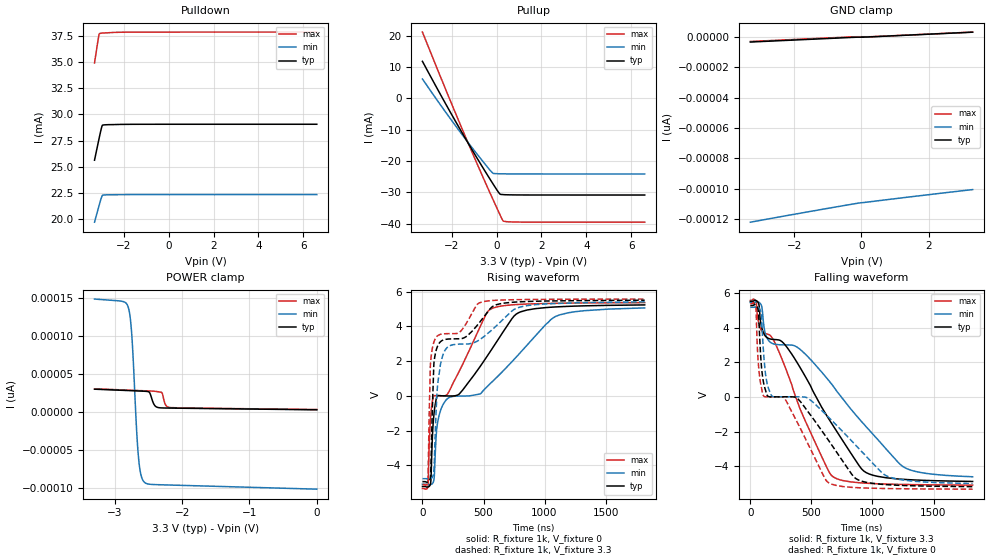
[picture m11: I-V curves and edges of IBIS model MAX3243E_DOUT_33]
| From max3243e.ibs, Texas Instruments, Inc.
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[Model]   MAX3243E_DOUT_33
Model_type  3-state
Enable   Active-High
Vref =   0
Rref =   3000
Cref =   150p
Vmeas =   1.5
| variable   typ   min   max
C_comp   3.62pF   2.98pF   4.25pF
| C_pullup   4.04pF   3.07pF   5.16pF
| C_pulldown   3.89pF   2.76pF   5.21pF
| C_tri-state   3.62pF   2.98pF   4.25pF
[Temperature Range]   40   100   -40
| Ambient temperature   25   85   -40
[Voltage range]   3.3   3   3.6
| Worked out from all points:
|   slope of the pullup table from 0 to 0.495 V, typ, clamps not added: 285 ohm
|   rising waveform, R_fixture 1k, V_fixture 0: 20-80 % time 533ns typ, 764ns min, 370ns max; typ from -5.23 V to 5.24 V
|   falling waveform, R_fixture 1k, V_fixture 3.3: 20-80 % time 648ns typ, 926ns min, 377ns max; typ from 5.53 V to -4.89 V
|   rising waveform, R_fixture 1k, V_fixture 3.3: 20-80 % time 285ns typ, 394ns min, 70.2ns max; typ from -4.95 V to 5.51 V
|   falling waveform, R_fixture 1k, V_fixture 0: 20-80 % time 619ns typ, 784ns min, 449ns max; typ from 5.29 V to -5.19 V
[GND Clamp]
| MAX3243E_DOUT_33
|   Voltage   I(typ)   I(min)   I(max)
-3.3V     -3.406pA   -122.2pA   -3.03pA
-1.41V    -1.49pA    -114.6pA   -1.116pA
-280mV    -348.5fA   -110.3pA   22.25fA
-95mV     -205.4fA   -109.6pA   87.86fA
75mV      -166.9fA   -109.2pA   91.62fA
320mV     65.63fA    -108.5pA   149.5fA
2.065V    1.838pA    -103.8pA   1.908pA
3.3V      3.096pA    -100.7pA   3.158pA
[POWER Clamp]
| MAX3243E_DOUT_33
|   Voltage   I(typ)   I(min)   I(max)
-3.3V     30.28pA    149pA      30.79pA
-2.875V   28.75pA    145.7pA    29.3pA
-2.795V   28.46pA    137pA      29.01pA
-2.77V    28.37pA    124.6pA    28.93pA
-2.745V   28.28pA    99.48pA    28.84pA
-2.675V   28.03pA    -23.88pA   28.59pA
-2.645V   27.92pA    -61.61pA   28.49pA
-2.61V    27.78pA    -82.83pA   28.36pA
-2.555V   27.54pA    -92.73pA   28.17pA
-2.335V   5.787pA    -95.6pA    26.65pA
-2.18V    5.387pA    -96pA      6.119pA
-48.03fV  3.096pA    -101.4pA   3.463pA
[Pulldown]
| MAX3243E_DOUT_33
|   Voltage   I(typ)   I(min)   I(max)
-3.3V     25.64mA    19.73mA    34.9mA
-3.155V   27.12mA    20.86mA    36.91mA
-3.12V    27.47mA    21.13mA    37.37mA
-3.095V   27.72mA    21.33mA    37.66mA
-3.075V   27.92mA    21.48mA    37.71mA
-3.02V    28.45mA    21.89mA    37.74mA
-2.965V   28.9mA     22.21mA    37.76mA
-2.95V    28.97mA    22.28mA    37.76mA
-2.905V   29mA       22.32mA    37.77mA
-2.335V   29.04mA    22.35mA    37.83mA
-1.555V   29.06mA    22.36mA    37.85mA
6.6V      29.07mA    22.36mA    37.85mA
[Pullup]
| MAX3243E_DOUT_33
|   Voltage   I(typ)   I(min)   I(max)
-3.3V     11.86mA    6.215mA    21.2mA
-1.69V    -9.033mA   -10.05mA   -7.06mA
-970mV    -17.85mA   -16.85mA   -19.17mA
-290mV    -25.8mA    -22.93mA   -30.21mA
-140mV    -27.5mA    -23.97mA   -32.59mA
135mV     -30.42mA   -24.08mA   -36.88mA
300mV     -30.74mA   -24.1mA    -39.19mA
1.16V     -30.86mA   -24.14mA   -39.53mA
6.6V      -30.87mA   -24.15mA   -39.56mA
[Ramp]
| MAX3243E_DOUT_33
| variable   typ   min   max
dV/dt_r   6.30/5.33E-07   6.12/7.64E-07   6.45/3.69E-07
dV/dt_f   6.29/6.55E-07   6.09/9.28E-07   6.46/3.82E-07
R_load = 1k
[Rising Waveform]
| MAX3243E_DOUT_33
R_fixture =   1k
C_fixture =   0
L_fixture =   0
V_fixture =   0
V_fixture_min = 0
V_fixture_max = 0
|   Time   V(typ)   V(min)   V(max)
0s        -5.226V    -5.098V    -5.343V
45.7ns    -5.252V    -5.123V    -5.181V
66.8ns    -5.036V    -5.114V    -1.248V
88.9ns    -1.5V      -4.976V    -69.7mV
118.4ns   -55.53mV   -1.824V    3.632mV
167.2ns   -1.325mV   -525.3mV   -7.684mV
545.8ns   2.454V     643.1mV    4.94V
769.1ns   4.719V     2.245V     5.264V
1.093us   5.128V     4.589V     5.336V
1.82us    5.244V     5.071V     5.375V
[Falling Waveform]
| MAX3243E_DOUT_33
R_fixture =   1k
C_fixture =   0
L_fixture =   0
V_fixture =   3.3
V_fixture_min = 3
V_fixture_max = 3.6
|   Time   V(typ)   V(min)   V(max)
0s        5.527V     5.458V     5.585V
46.1ns    5.576V     5.524V     5.526V
65.8ns    5.438V     5.491V     4.369V
87.7ns    4.188V     5.334V     3.887V
156.1ns   3.365V     3.207V     3.595V
305.8ns   2.816V     3.009V     1.338V
671.7ns   -1.598V    688.3mV    -4.585V
929.6ns   -4.289V    -1.569V    -4.981V
1.252us   -4.764V    -4.038V    -5.06V
1.82us    -4.886V    -4.616V    -5.099V
[Rising Waveform]
| MAX3243E_DOUT_33
R_fixture =   1k
C_fixture =   0
L_fixture =   0
V_fixture =   3.3
V_fixture_min = 3
V_fixture_max = 3.6
|   Time   V(typ)   V(min)   V(max)
0s        -4.949V    -4.778V    -5.116V
45.3ns    -4.965V    -4.8V      -4.826V
65.9ns    -4.645V    -4.781V    1.851V
93.1ns    1.769V     -4.361V    3.085V
123.2ns   2.854V     539.6mV    3.457V
201.1ns   3.268V     2.779V     3.585V
310.1ns   3.292V     2.983V     3.703V
466ns     4.217V     3.226V     5.363V
771.3ns   5.411V     5.055V     5.546V
1.82us    5.511V     5.418V     5.58V
[Falling Waveform]
| MAX3243E_DOUT_33
R_fixture =   1k
C_fixture =   0
L_fixture =   0
V_fixture =   0
V_fixture_min = 0
V_fixture_max = 0
|   Time   V(typ)   V(min)   V(max)
0s        5.287V     5.186V     5.388V
44.7ns    5.318V     5.239V     5.174V
64.4ns    5.013V     5.189V     2.042V
103.9ns   995.7mV    3.01V      112.4mV
174.7ns   2.007mV    66.51mV    7.519mV
282.9ns   8.931mV    6.894mV    -105.9mV
633.1ns   -2.438V    -1.122V    -4.922V
859.4ns   -4.697V    -2.767V    -5.241V
1.118us   -5.074V    -4.575V    -5.297V
1.82us    -5.189V    -5.01V     -5.333V
